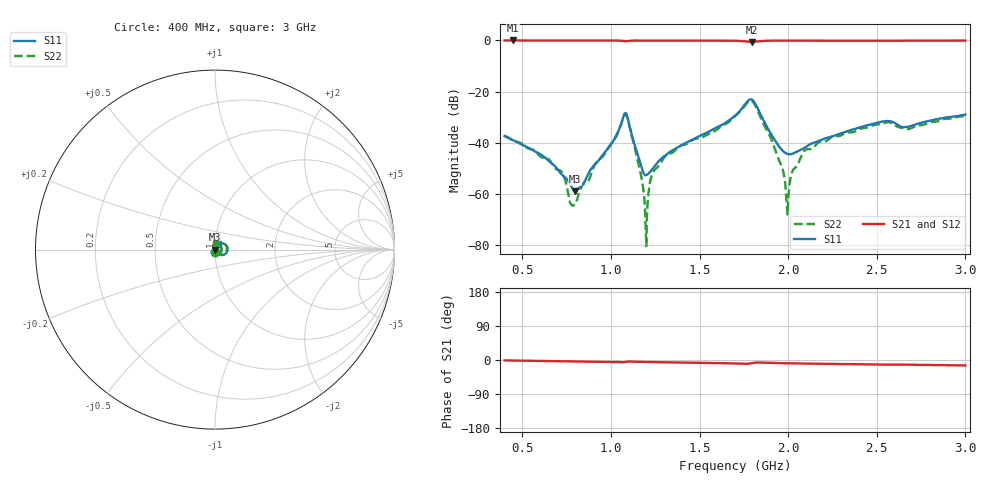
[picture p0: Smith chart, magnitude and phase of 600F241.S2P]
!  American Technical Ceramics  Date:  12/6/06
!  One Norden Lane
!  Huntington Station,  NY.  11746-2102
!  Tel:  (631) 622-4700  Fax:  (631) 622-4748
!  Part Number  600F241  Mounting Orientation: Horizontal
!  Description: Ultra Low ESR Microwave capacitors
!  Application: Coupling, Bypass, Tuning, DC Block
!  Filters, Matching
# GHZ S DB R 50
! Freq  |S11|  S11 Ph  |S21|  S21 Ph  |S12|  S12 Ph  |S22|  S22 Ph
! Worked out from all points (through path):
!   801 points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, 400 MHz to 3 GHz, reference 50 ohm
!   highest |S21| = 0.00 dB at 446 MHz (marker M1); lowest = -0.6 dB at 1.794 GHz (marker M2)
!   group delay of S21, straight-line fit = 13.4 ps
!   lowest |S11| = -58.9 dB at 797 MHz (marker M3), VSWR 1.00, Z = 50.1 - j0.0389 ohm
!   |S11| at or under -10 dB: start of sweep to end of sweep
!   |S22| runs from -80.4 to -23.5 dB; largest |S21 - S12| = 0.0025
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0.4  -37.36 -90.0  -0.01 -1.1  -0.01 -1.1  -37.28 -89.9
0.446  -38.88 -89.2  0.00 -1.4  -0.01 -1.4  -39.10 -91.0
0.719  -52.11 -73.4  -0.01 -3.1  -0.01 -3.1  -51.19 -97.3
0.774  -56.81 -51.7  -0.01 -3.4  -0.01 -3.5  -63.92 -110.2
0.797  -58.94 -20.1  -0.01 -3.6  -0.01 -3.6  -64.06 -136.9
0.836  -56.72 26.6  -0.01 -3.8  -0.01 -3.8  -56.95 116.4
1.079  -28.43 9.3  -0.32 -5.5  -0.30 -5.5  -28.77 18.6
1.161  -46.76 -55.8  -0.03 -5.0  -0.02 -5.0  -49.73 -70.5
1.196  -52.70 -8.1  -0.02 -5.3  -0.01 -5.3  -73.71 -92.0
1.206  -52.41 6.8  -0.02 -5.4  0.00 -5.4  -64.38 115.3
1.232  -50.41 34.3  -0.02 -5.6  0.00 -5.6  -52.37 97.0
1.268  -47.40 51.7  -0.02 -5.8  0.00 -5.9  -49.19 93.9
1.7  -29.43 56.6  -0.10 -9.3  -0.09 -9.3  -29.65 72.1
1.794  -23.07 -3.9  -0.62 -8.3  -0.61 -8.4  -23.64 2.2
1.915  -37.86 -50.6  -0.07 -7.8  -0.06 -7.9  -40.25 -70.6
1.967  -43.00 -27.7  -0.05 -8.4  -0.04 -8.5  -49.76 -65.5
1.996  -44.35 -7.7  -0.04 -8.7  -0.03 -8.7  -68.05 -172.7
2.028  -44.16 14.2  -0.04 -8.9  -0.02 -9.0  -50.57 86.3
2.136  -40.21 47.2  -0.03 -9.7  -0.02 -9.7  -42.26 92.4
2.568  -31.50 46.0  -0.10 -12.3  -0.09 -12.3  -31.96 69.2
2.678  -33.71 53.6  -0.07 -12.4  -0.05 -12.4  -34.64 73.6
3  -28.98 63.5  -0.05 -14.4  -0.04 -14.4  -29.44 79.4
